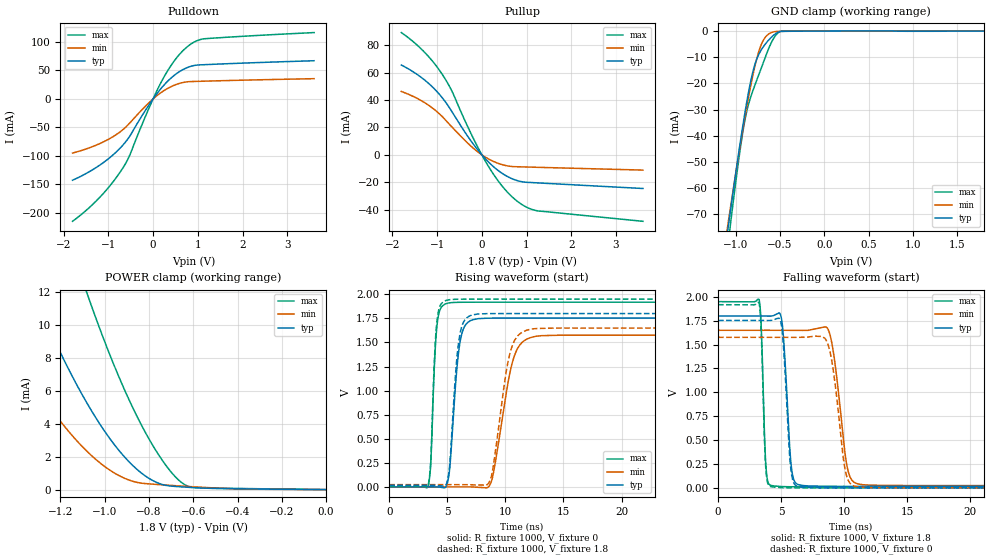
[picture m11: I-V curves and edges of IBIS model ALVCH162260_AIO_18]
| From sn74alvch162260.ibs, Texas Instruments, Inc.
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[Model]   ALVCH162260_AIO_18
Model_type  I/O
Vinl=0.5775
Vinh=1.2675
Enable   Active-Low
Vref =   0
Rref =   1000
Cref =   30p
Vmeas =   0.9
| variable   typ   min   max
C_comp   8.83pF   7.78pF   9.62pF
| C_pullup   9.93pF   8.30pF   10.76pF
| C_pulldown   13.53pF   10.28pF   17.43pF
| C_tri-state   8.83pF   7.78pF   9.62pF
[Temperature Range]   40   100   -40
| Ambient temperature   25   85   -40
[Voltage range]   1.8   1.65   1.95
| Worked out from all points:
|   slope of the pulldown table from 0 to 0.27 V, typ, clamps not added: 10.2 ohm
|   slope of the pullup table from 0 to 0.27 V, typ, clamps not added: 30.2 ohm
|   GND clamp passes 1 mA (typ) near -0.55 V on its own axis
|   POWER clamp passes 1 mA (typ) near -0.83 V on its own axis
|   rising waveform, R_fixture 1000, V_fixture 0: 20-80 % time 662ps typ, 1.32ns min, 387ps max; typ from 0 V to 1.75 V
|   falling waveform, R_fixture 1000, V_fixture 1.8: 20-80 % time 455ps typ, 832ps min, 270ps max; typ from 1.8 V to 0.016 V
|   rising waveform, R_fixture 1000, V_fixture 1.8: 20-80 % time 623ps typ, 1.15ns min, 377ps max; typ from 0.016 V to 1.8 V
|   falling waveform, R_fixture 1000, V_fixture 0: 20-80 % time 443ps typ, 827ps min, 264ps max; typ from 1.75 V to 0 V
[GND Clamp]
| ALVCH162260_AIO_18
|   Voltage   I(typ)   I(min)   I(max)
-1.8V     -267.7mA   -247.3mA   -300.9mA
-1.09V    -76.1mA    -74.2mA    -82.32mA
-1.075V   -72.37mA   -70.82mA   -78.1mA
-1.055V   -67.46mA   -66.36mA   -72.53mA
-920mV    -36.17mA   -37.65mA   -38.59mA
-875mV    -26.98mA   -28.88mA   -30.56mA
-820mV    -17.47mA   -19.08mA   -24.08mA
-720mV    -7.652mA   -5.864mA   -14.89mA
-620mV    -3.141mA   -959.9uA   -6.029mA
-555mV    -1.142mA   -210.2uA   -1.921mA
-485mV    -97.9uA    -108.2uA   -133.2uA
1.8V      63.53pA    9.524uA    -22.72uA
[POWER Clamp]
| ALVCH162260_AIO_18
|   Voltage   I(typ)   I(min)   I(max)
-1.8V     29.94mA    18.79mA    48.32mA
-1.545V   19.69mA    11.65mA    33.78mA
-1.31V    11.56mA    6.211mA    21.83mA
-1.19V    8.026mA    3.974mA    16.4mA
-1.08V    5.242mA    2.322mA    11.91mA
-1.065V   4.9mA      2.13mA     11.33mA
-925mV    2.204mA    777.7uA    6.495mA
-850mV    1.177mA    426.3uA    4.328mA
-770mV    462.3uA    318uA      2.392mA
-695mV    208uA      249.8uA    983.5uA
-635mV    150uA      199.3uA    273.7uA
-16.28fV  63.53pA    285.3pA    36.64pA
[Pulldown]
| ALVCH162260_AIO_18
|   Voltage   I(typ)   I(min)   I(max)
-1.8V     -142.5mA   -94.94mA   -214.6mA
-1.19V    -116mA     -78.24mA   -172.4mA
-930mV    -100.5mA   -67.79mA   -148.9mA
-690mV    -82.3mA    -54.81mA   -122.9mA
-535mV    -66.97mA   -43.32mA   -101mA
-105mV    -12.13mA   -7.634mA   -18.73mA
200mV     20.41mA    12.38mA    32.16mA
490mV     42.45mA    24.65mA    68.46mA
785mV     55.72mA    30.25mA    92.88mA
970mV     59.35mA    30.84mA    101.8mA
1.155V    60.2mA     31.26mA    105.7mA
3.6V      67.09mA    35.62mA    116.5mA
[Pullup]
| ALVCH162260_AIO_18
|   Voltage   I(typ)   I(min)   I(max)
-1.8V     65.54mA    46.25mA    89.25mA
-1.32V    55.67mA    38.89mA    76.19mA
-1.11V    49.72mA    34.29mA    68.65mA
-920mV    43.05mA    29.01mA    60.43mA
-685mV    32.34mA    20.89mA    47.55mA
-250mV    10.47mA    6.526mA    16.03mA
115mV     -4.131mA   -2.38mA    -6.642mA
450mV     -13.44mA   -7.131mA   -22.64mA
790mV     -18.81mA   -8.709mA   -33.84mA
1.02V     -20.1mA    -8.918mA   -38.54mA
1.25V     -20.5mA    -9.124mA   -40.92mA
3.6V      -24.58mA   -11.14mA   -48.53mA
[Ramp]
| ALVCH162260_AIO_18
| variable   typ   min   max
dV/dt_r   1.06/6.69E-10   0.95/1.32E-09   1.16/3.98E-10
dV/dt_f   1.09/4.68E-10   1.00/8.58E-10   1.18/2.77E-10
R_load = 1000
[Rising Waveform]
| ALVCH162260_AIO_18
R_fixture =   1000
C_fixture =   0
L_fixture =   0
V_fixture =   0
V_fixture_min = 0
V_fixture_max = 0
|   Time   V(typ)   V(min)   V(max)
0s        343.1pV    1.757nV    237.2pV
3.35ns    712.2uV    -78.37uV   8.114mV
4.1ns     -105.1uV   -77.37uV   1.662V
4.935ns   13.88mV    477.2uV    1.904V
6.07ns    1.486V     241.4uV    1.917V
7.19ns    1.736V     -911.7uV   1.918V
8.755ns   1.752V     43.42mV    1.918V
10.61ns   1.753V     1.298V     1.918V
12.23ns   1.753V     1.553V     1.918V
50ns      1.753V     1.576V     1.918V
[Falling Waveform]
| ALVCH162260_AIO_18
R_fixture =   1000
C_fixture =   0
L_fixture =   0
V_fixture =   1.8
V_fixture_min = 1.65
V_fixture_max = 1.95
|   Time   V(typ)   V(min)   V(max)
0s        1.8V       1.65V      1.95V
3.255ns   1.8V       1.65V      1.972V
3.79ns    1.799V     1.65V      240mV
4.205ns   1.798V     1.65V      25.13mV
5.05ns    1.758V     1.65V      13.92mV
5.795ns   242.3mV    1.649V     11.52mV
6.41ns    32.04mV    1.649V     11.21mV
8.775ns   16.24mV    1.645V     11.08mV
11.07ns   15.91mV    41.91mV    11.07mV
50ns      15.9mV     23.5mV     11.07mV
[Rising Waveform]
| ALVCH162260_AIO_18
R_fixture =   1000
C_fixture =   0
L_fixture =   0
V_fixture =   1.8
V_fixture_min = 1.65
V_fixture_max = 1.95
|   Time   V(typ)   V(min)   V(max)
0s        15.9mV     23.5mV     11.07mV
3.35ns    16.48mV    23.44mV    20.72mV
4.09ns    15.3mV     23.46mV    1.702V
4.905ns   25.84mV    23.89mV    1.937V
6.01ns    1.532V     23.09mV    1.949V
7.085ns   1.784V     22.09mV    1.95V
8.715ns   1.8V       77.02mV    1.95V
10.36ns   1.8V       1.371V     1.95V
11.88ns   1.8V       1.629V     1.95V
50ns      1.8V       1.65V      1.95V
[Falling Waveform]
| ALVCH162260_AIO_18
R_fixture =   1000
C_fixture =   0
L_fixture =   0
V_fixture =   0
V_fixture_min = 0
V_fixture_max = 0
|   Time   V(typ)   V(min)   V(max)
0s        1.753V     1.576V     1.918V
3.255ns   1.753V     1.576V     1.936V
3.77ns    1.752V     1.576V     237.5mV
4.13ns    1.752V     1.576V     14.5mV
5.03ns    1.703V     1.576V     2.573mV
5.745ns   232.5mV    1.576V     408.9uV
6.325ns   15.1mV     1.576V     129.5uV
8.675ns   275.1uV    1.516V     4.301uV
10.87ns   12.82uV    15.34mV    1.18uV
50ns      356nV      789.5nV    157.3nV
